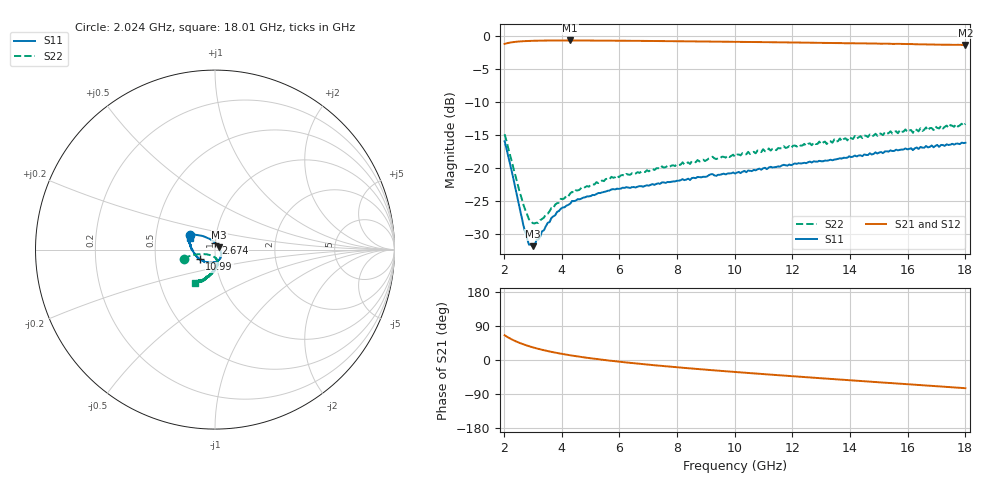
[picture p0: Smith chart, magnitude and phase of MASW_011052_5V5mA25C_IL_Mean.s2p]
! MA-COM, USA
! Part Number: MASW-011052
! Data: 29-03-2013
! Bias Condition:
!  Insertion Loss in ON stage Antenna (1) to RFin (2)
!  Forward Bias (series Diode and Shunt Diode) I = 5 mA
!  Reverse Bias Voltage V = -5V
!  Temp: 25C
!  VAR RecID: Mean
# HZ S DB R 50
! F n11x n11y n21x n21y n12x n12y n22x n22y
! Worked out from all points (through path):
!   247 points, 2.024 GHz to 18.01 GHz, reference 50 ohm
!   highest |S21| = -0.60 dB at 4.298 GHz (marker M1); lowest = -1.3 dB at 18.01 GHz (marker M2)
!   lowest |S11| = -31.8 dB at 2.999 GHz (marker M3), VSWR 1.05, Z = 52.3 + j1.25 ohm
!   |S11| at or under -10 dB: start of sweep to end of sweep
!   |S22| runs from -28.4 to -13.2 dB; largest |S21 - S12| = 0.0081
!   S11 on the Smith chart (normalised r, x): 2.024 GHz: 0.75, +0.13; 2.674 GHz: 1.00, +0.07; 10.99 GHz: 0.84, -0.09; 18.01 GHz: 0.75, +0.10
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2.0242e9  -15.90 148.5  -1.12 65.3  -1.11 65.3  -14.83 -164.0
2.3491e9  -22.04 123.9  -0.84 51.6  -0.83 51.6  -20.31 -164.6
2.674e9  -28.64 87.9  -0.71 41.4  -0.72 41.4  -25.50 -150.3
2.8689e9  -31.59 53.3  -0.68 36.4  -0.68 36.4  -27.75 -132.7
2.9989e9  -31.82 27.7  -0.66 33.4  -0.66 33.5  -28.33 -120.8
3.1938e9  -30.83 -0.2  -0.64 29.4  -0.64 29.4  -28.30 -104.0
3.6486e9  -27.54 -33.4  -0.61 21.4  -0.62 21.5  -26.02 -84.8
4.2984e9  -25.38 -56.7  -0.60 12.4  -0.61 12.5  -23.82 -76.2
4.6882e9  -24.60 -64.1  -0.61 7.9  -0.62 8.0  -22.96 -77.6
5.7278e9  -23.22 -84.2  -0.64 -2.2  -0.64 -2.1  -21.29 -79.4
7.3522e9  -22.29 -106.7  -0.69 -14.8  -0.70 -14.7  -19.98 -86.6
1.0081e10  -20.66 -137.1  -0.81 -32.0  -0.82 -31.9  -17.93 -95.3
1.0991e10  -20.01 -148.0  -0.86 -37.2  -0.87 -37.0  -17.12 -97.6
1.2745e10  -18.96 -163.3  -0.95 -46.8  -0.96 -46.6  -16.09 -103.8
1.32e10  -18.86 -166.2  -0.97 -49.2  -0.98 -49.0  -16.32 -105.7
1.346e10  -18.68 -170.0  -1.00 -50.6  -0.99 -50.3  -15.62 -106.1
1.5409e10  -17.28 174.1  -1.11 -60.8  -1.14 -60.7  -14.38 -112.7
1.6189e10  -17.25 169.2  -1.16 -64.9  -1.20 -64.8  -14.62 -115.0
1.6254e10  -16.97 168.0  -1.18 -65.2  -1.18 -65.1  -14.06 -114.0
1.6904e10  -16.82 164.5  -1.21 -68.7  -1.25 -68.4  -14.20 -117.7
1.6968e10  -16.60 163.9  -1.21 -68.9  -1.25 -68.8  -13.66 -117.3
1.8008e10  -16.12 155.1  -1.30 -74.4  -1.28 -74.2  -13.23 -120.2
